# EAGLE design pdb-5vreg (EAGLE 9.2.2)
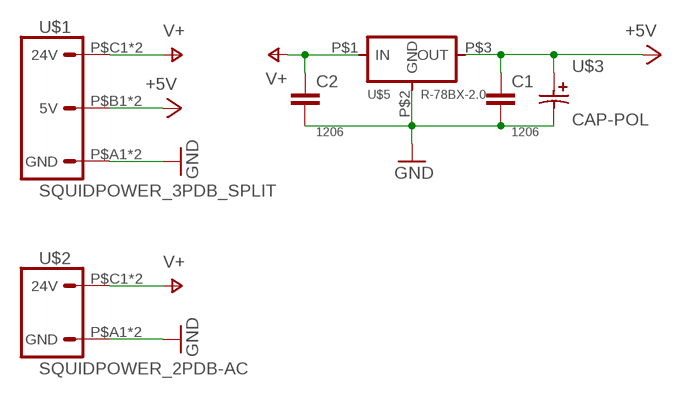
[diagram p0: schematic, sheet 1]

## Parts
C1  CAP1206  [1206]
C2  CAP1206  [1206]
U$1  SQUIDPOWER_3PDB_SPLIT  [PDBCONN_3]
U$2  SQUIDPOWER_2PDB-AC  [PDBCONN_AC]
U$3  CAP-POL  [SMD-ELEC-CAP]
U$5  R-78BX-2.0  [R-78BX-2.0]

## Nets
+5V: C1.1 U$1.P$B1(5V) U$1.P$B2(5V) U$3.A U$5.P$3(OUT)
GND: C1.2 C2.2 U$1.P$A1(GND) U$1.P$A2(GND) U$2.P$A1(GND) U$2.P$A2(GND) U$3.C U$5.P$2(GND)
V+: C2.1 U$1.P$C1(24V) U$1.P$C2(24V) U$2.P$C1(24V) U$2.P$C2(24V) U$5.P$1(IN)

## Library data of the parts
C1 C2 = passives:CAP: Capacitor; PACKAGE: 1206
U$1 = connector:SQUIDPOWER_3
U$2 = connector:SQUIDPOWER_2
U$3 = passives:CAP-POL
U$5 = power:R-78BX-2.0

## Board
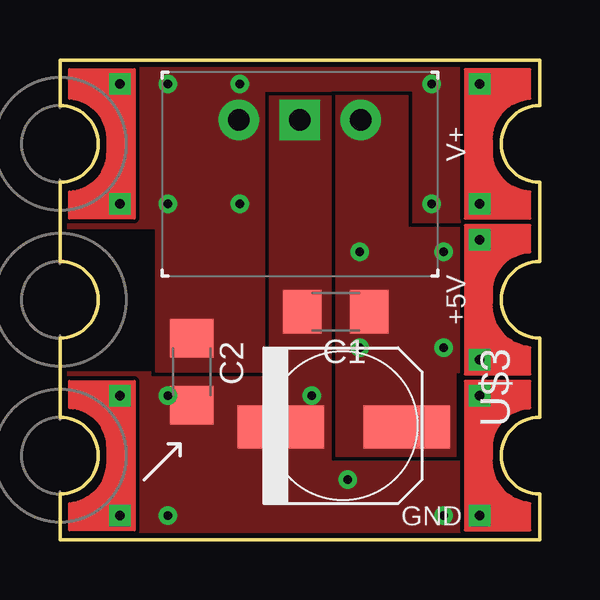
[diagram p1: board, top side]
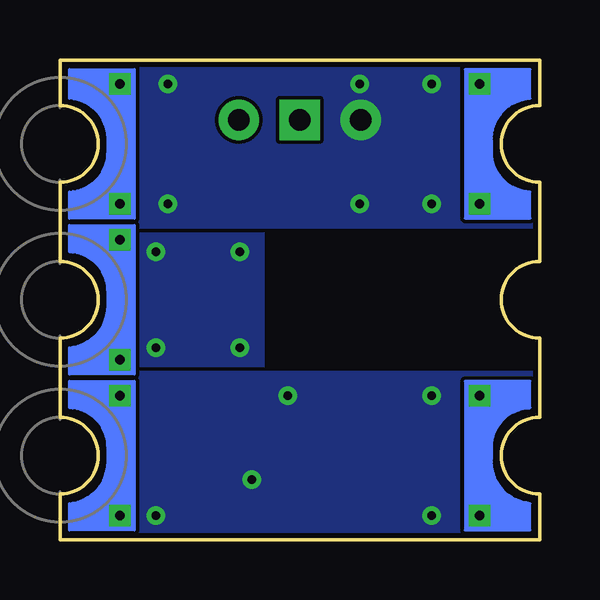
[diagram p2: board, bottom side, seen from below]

Size 20 x 20 mm. Coordinates in mm from the lower left corner, seen from the top.
Outline: 0,5.1 0,8.4 arc90 1.6,10 arc90 0,11.6 0,14.9 arc90 1.6,16.5 arc90 0,18.1 0,20 20,20 20,18.1 arc90 18.4,16.5 arc90 20,14.9 20,11.6 arc90 18.4,10 arc90 20,8.4 20,5.1 arc90 18.4,3.5 arc90 20,1.9 20,0 0,0 0,1.9 arc90 1.6,3.5 arc90 0,5.1
Copper layers (1*16): Top 0.035mm / dielectric 1.5mm / Bottom 0.035mm
Design rules "default *": minimum track width 6mil, minimum drill 0.35mm, track to track 6mil, track to pad 6mil, pad to pad 6mil, via to via 6mil, smd to smd 6mil, copper to edge 8mil, drill to drill 6mil, minimum pad ring 10mil, minimum via ring 8mil, stop-mask expansion 4mil, vias tented up to drill 30mil, thermal gap 10mil

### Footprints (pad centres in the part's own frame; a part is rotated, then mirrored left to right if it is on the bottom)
1206 = smd 1.6 x 1.8: 1 -1.4,0; 2 1.4,0
PDBCONN_3 = drill 0.4 square: P$A1 2.5,-9; P$A2 2.5,-4; P$B1 2.5,-2.5; P$B2 2.5,2.5; P$C1 2.5,4; P$C2 2.5,9
PDBCONN_AC = drill 0.4 square: P$A1 2.5,-9; P$A2 2.5,-4; P$C1 2.5,4; P$C2 2.5,9
SMD-ELEC-CAP = smd 1.8 x 3.6: A 3.3,5.95; C 3.3,0.7
R-78BX-2.0 = drill 0.9 pad 1.676: P$1 -2.54,0; P$3 2.54,0 | drill 0.9 pad 1.676 square: P$2 0,0

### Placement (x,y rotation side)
C1  11.5,9.5 180 top
C2  5.5,7 270 top
U$1  20,10 0 bottom
U$2  0,10 0 top
U$3  8.5,8 270 top
U$5  10,17.5 0 top

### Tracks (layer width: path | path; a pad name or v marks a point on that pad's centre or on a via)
+5V  (via drill 0.35)
  other vias: 12.5,8 12.5,12 16,12 16,8
  pour Bottom (rank 6, no thermals): 11.5,13 24,13 24,7 11.5,7
  pour Top (rank 4, no thermals): 11.5,18.5 11.5,7 21,7 21,13 14.5,13 14.5,18.5
  pour Top (rank 3, no thermals): 11.5,7.5 11.5,3.5 16.5,3.5 16.5,7.5
GND  (via drill 0.35)
  other vias: 16,1 12,2.5 10.5,6 4.5,6 4.5,1
  pour Bottom (rank 2, no thermals): -3.5,7 23.5,7 23.5,-1 -3.5,-1
  pour Top (rank 5, no thermals): 11.5,18.5 11.5,7 21,7 21,-0.5 -1,-0.5 -1,7 8.5,7 8.5,18.5
V+  (via drill 0.35)
  other vias: 7.5,14 15.5,14 15.5,19 7.5,19 4.5,14 4.5,19
  pour Bottom (rank 2, no thermals): -3.5,13 23.5,13 23.5,21 -3.5,21
  pour Top (rank 4, no thermals): 8.5,19 8.5,7 4,7 4,19
  pour Top (rank 6, no thermals): 21,13 21,20.5 -1,20.5 -1,13

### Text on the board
tPlace: V+ | +5V | GND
